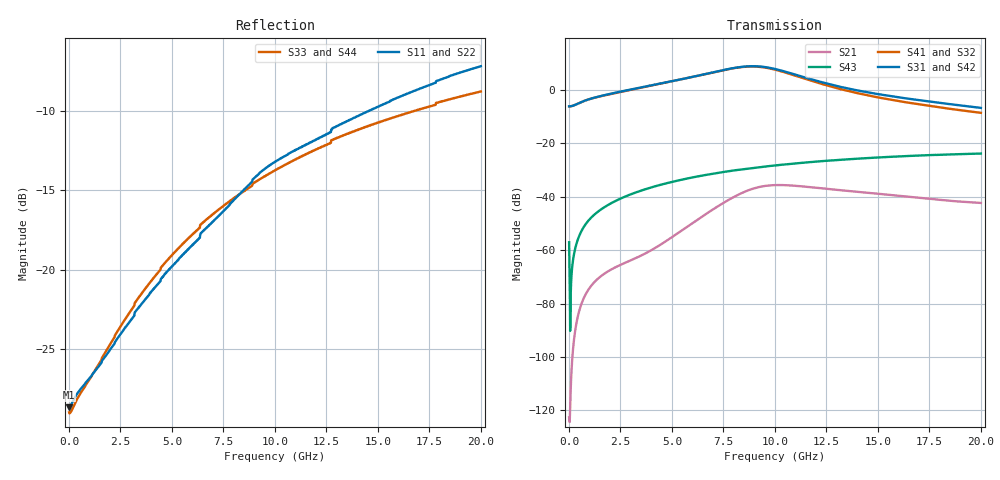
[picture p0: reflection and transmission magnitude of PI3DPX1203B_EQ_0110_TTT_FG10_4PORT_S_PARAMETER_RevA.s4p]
! NPort=4 DATA=2000 NOISE=0 GROUPDELAY=0 COMPLEX_DATAFORMAT=POLAR
! NumOfBlock=1 NumOfParam=0
! .MODEL Smodel S TSTONEFILE=PI3DPX1203B_EQ_0110_TTT_FG10_4PORT_S_PARAMETER_RevA.s4p TYPE=S
!  -- The above .MODEL line can be used for the S element in the netlist.
! The s parameter is extracted from the linear redriver, it is not bi-directional; only s(4,1)s(4,2) and s(3,1)s(3,2)
! should be the insertion loss
!Port definition:
!Port1 = input+
!Port2 = input-
!Port3 = output+
!Port4 = output-
# Hz S MA R  50
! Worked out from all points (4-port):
!   2000 points, 10 MHz to 20 GHz, reference 50 ohm
!   strongest paths, dB at 10 MHz, 5.01 GHz, 10.01 GHz, 15.01 GHz, 20 GHz:
!     S31: -6.2, 3.3, 7.8, -1.6, -6.7
!     S42: -6.2, 3.3, 7.8, -1.6, -6.7
!     S41: -6.2, 3.2, 7.6, -2.8, -8.6
!     S32: -6.2, 3.2, 7.6, -2.8, -8.6
!     S43: -57.1, -34.4, -28.3, -25.3, -23.8
!     S21: -122.7, -55.1, -35.6, -38.9, -42.3
!   lowest |S11| = -28.6 dB at 10 MHz (marker M1), VSWR 1.08, Z = 46.4 - j0.0306 ohm
!   |S11| at or under -10 dB: start of sweep to 14.58 GHz
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1e7  0.03701 -179.5  7.338e-07 10.6  0 0.0  0 0.0
     7.338e-07 10.6  0.03701 -179.5  0 0.0  0 0.0
     0.4917 -0.1  0.4917 179.9  0.03566 178.2  0.001403 -77.8
     0.4917 179.9  0.4917 -0.1  0.001403 -77.8  0.03566 178.2
1.56e9  0.05087 -144.9  0.0003264 116.6  4.972e-12 74.2  4.731e-11 115.3
        0.0003264 116.6  0.05087 -144.9  4.731e-11 115.3  4.972e-12 74.2
        0.7704 8.3  0.7636 -171.7  0.05186 -142.3  0.005788 82.9
        0.7636 -171.7  0.7704 8.3  0.005788 82.9  0.05186 -142.3
6.07e9  0.1212 -110.8  0.003358 145.8  1.61e-08 -118.0  1.429e-07 66.8
        0.003358 145.8  0.1212 -110.8  1.428e-07 66.7  1.61e-08 -118.0
        1.778 -44.1  1.776 137.7  0.1306 -117.0  0.02326 64.8
        1.776 137.7  1.778 -44.1  0.02326 64.8  0.1306 -117.0
8.46e9  0.1777 -105.5  0.01206 108.5  3.789e-07 156.9  1.045e-06 17.4
        0.01205 108.5  0.1777 -105.5  1.044e-06 17.4  3.788e-07 156.9
        2.721 -100.4  2.692 81.1  0.1763 -115.9  0.03281 52.5
        2.693 81.1  2.72 -100.4  0.03281 52.5  0.1763 -115.9
9.94e9  0.2173 -107.2  0.01649 65.4  1.218e-06 95.3  2.077e-06 -20.2
        0.01648 65.4  0.2173 -107.2  2.074e-06 -20.1  1.217e-06 95.3
        2.499 -148.9  2.429 32.5  0.2044 -116.3  0.03827 44.7
        2.43 32.5  2.497 -148.9  0.03827 44.7  0.2044 -116.3
1.21e10  0.2583 -108.9  0.01462 23.7  3.029e-06 30.2  3.834e-06 -48.0
         0.01462 23.8  0.2583 -108.9  3.834e-06 -47.8  3.03e-06 30.2
         1.454 164.9  1.354 -13.3  0.241 -117.5  0.04577 33.6
         1.355 -13.3  1.453 165.0  0.04577 33.6  0.241 -117.5
2e10  0.4369 -117.0  0.007613 -18.2  2.218e-05 -107.6  3.194e-05 -133.9
      0.007647 -18.4  0.437 -117.1  3.202e-05 -133.8  2.22e-05 -107.6
      0.461 79.6  0.3728 -85.2  0.3637 -123.9  0.06431 -7.1
      0.3722 -85.3  0.4614 79.7  0.06431 -7.1  0.3637 -123.9
